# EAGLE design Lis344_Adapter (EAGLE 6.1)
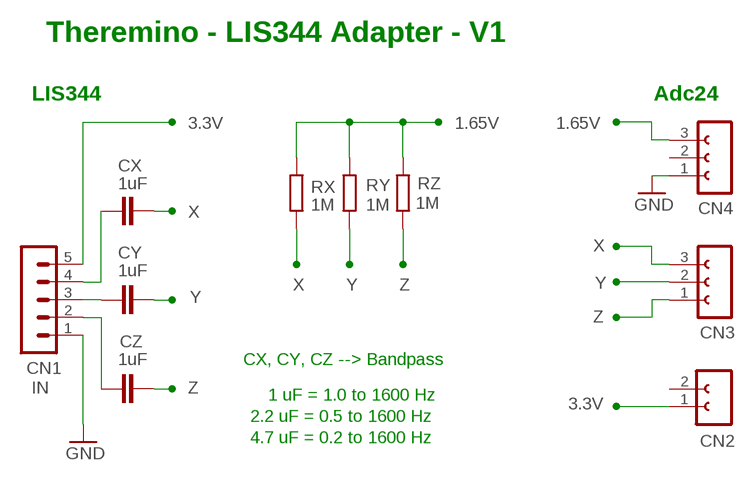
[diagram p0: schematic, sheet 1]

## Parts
CN1  IN  MA05-1  [MA05-1]
CN2  FE02-1L2  [FE02-1_L2]
CN3  FE03-1L3  [FE03-1_L3]
CN4  FE03-1L3  [FE03-1_L3]
CX  1uF  C-EUC0805  [C0805]
CY  1uF  C-EUC0805  [C0805]
CZ  1uF  C-EUC0805  [C0805]
RX  1M  R-EU_R0805  [R0805]
RY  1M  R-EU_R0805  [R0805]
RZ  1M  R-EU_R0805  [R0805]

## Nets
1.65V: CN4.3 RX.2 RY.2 RZ.2
3.3V: CN1.5 CN2.1
GND: CN1.1 CN4.1
N$13: CN1.3 CY.1
N$18: CN1.4 CX.1
N$99: CN1.2 CZ.1
X: CN3.3 CX.2 RX.1
Y: CN3.2 CY.2 RY.1
Z: CN3.1 CZ.2 RZ.1
Unconnected: CN2.2 CN4.2

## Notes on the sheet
- Theremino - LIS344 Adapter - V1
- LIS344 | Adc24
- CX, CY, CZ --> Bandpass
- 1 uF = 1.0 to 1600 Hz
- 2.2 uF = 0.5 to 1600 Hz
- 4.7 uF = 0.2 to 1600 Hz

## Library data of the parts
CN1 = 03-con-lstb-M:MA05-1: PIN HEADER
CN2 = 02-con-lsta-F:FE02-1: FEMALE HEADER
CN3 CN4 = 02-con-lsta-F:FE03-1: FEMALE HEADER
CX CY CZ = 00-LIVIO:C-EU: CAPACITOR, European symbol
RX RY RZ = 00-LIVIO:R-EU_: RESISTOR, European symbol

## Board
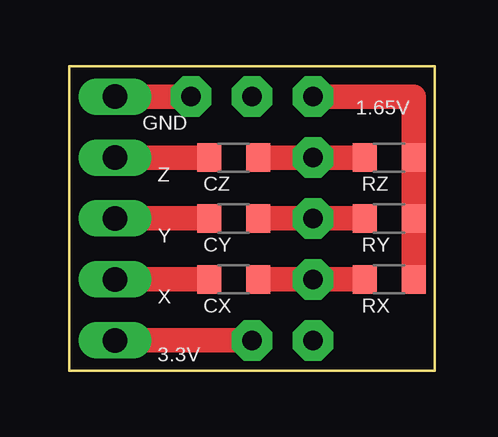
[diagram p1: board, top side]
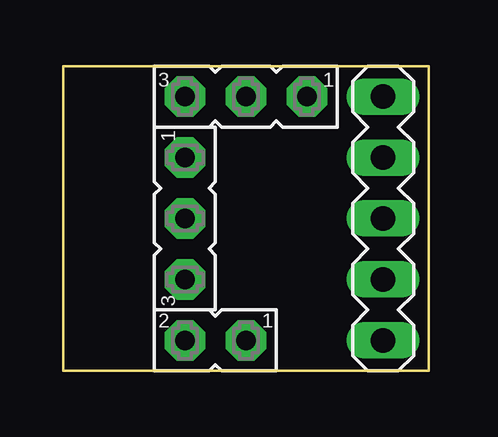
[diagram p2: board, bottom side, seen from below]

Size 15.24 x 12.7 mm. Coordinates in mm from the lower left corner, seen from the top.
Outline: 0,0 15.24,0 15.24,12.7 0,12.7 0,0
Copper layers (1*16): Top 0.035mm / dielectric 1.5mm / Bottom 0.035mm
Design rules: minimum track width 10mil, minimum drill 31mil, track to track 31mil, track to pad 31mil, pad to pad 31mil, via to via 31mil, smd to smd 31mil, copper to edge 31mil, drill to drill 8mil, minimum pad ring 5mil, minimum via ring 8mil, stop-mask expansion 4mil, vias tented up to drill 0mil, thermal gap 47mil

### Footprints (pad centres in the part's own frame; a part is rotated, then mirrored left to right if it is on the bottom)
MA05-1 = drill 1.016 long: 1 -5.08,0; 2 -2.54,0; 3 0,0; 4 2.54,0; 5 5.08,0
FE02-1_L2 = drill 0.813 pad 1.676 octagon: 1 -1.27,0; 2 1.27,0
FE03-1_L3 = drill 0.813 pad 1.676 octagon: 1 -2.54,0; 2 0,0; 3 2.54,0
C0805 = smd 1 x 1.2: 1 -1.016,0; 2 1.016,0
R0805 = smd 1 x 1.2: 1 -1.016,0; 2 1.016,0

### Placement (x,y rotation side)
CN1  1.91,6.35 270 bottom
CN2  8.89,1.27 180 bottom
CN3  10.16,6.35 270 bottom
CN4  7.62,11.43 180 bottom
CX  6.86,3.81 0 top
CY  6.86,6.35 0 top
CZ  6.86,8.89 0 top
RX  13.34,3.81 0 top
RY  13.34,6.35 0 top
RZ  13.34,8.89 0 top

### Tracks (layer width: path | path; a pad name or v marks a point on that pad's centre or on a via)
1.65V
  Top 1.016: CN4.3 14.35,11.43 RZ.2 RY.2 RX.2
3.3V
  Top 1.016: CN1.5 CN2.1
GND
  Top 1.016: CN1.1 CN4.1
N$13
  Top 1.016: CY.1 CN1.3
N$18
  Top 1.016: CX.1 CN1.4
N$99
  Top 1.016: CZ.1 CN1.2
X
  Top 1.016: CX.2 CN3.3 RX.1
Y
  Top 1.016: RY.1 CN3.2 CY.2
Z
  Top 1.016: CZ.2 CN3.1 RZ.1

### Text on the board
tNames: 1.65V | GND | Z | Y | X | 3.3V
